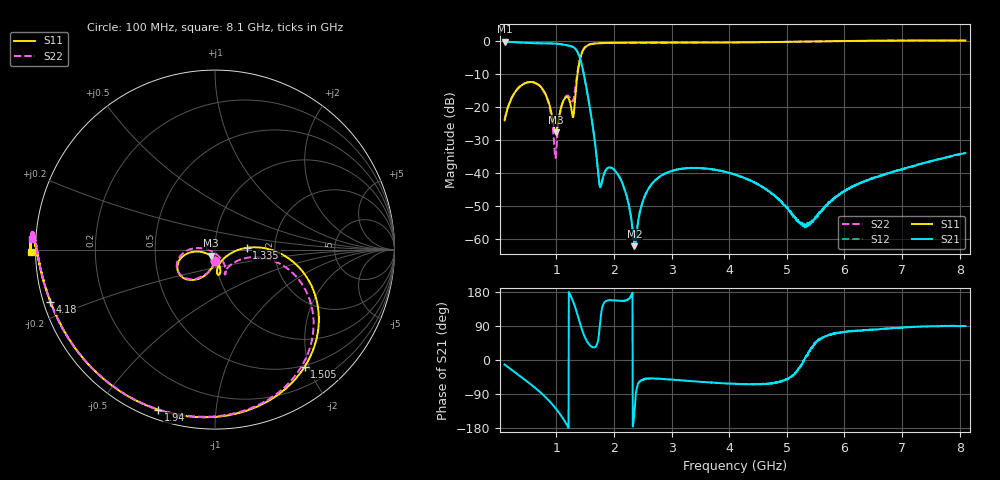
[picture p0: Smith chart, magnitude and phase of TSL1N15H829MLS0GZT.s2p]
! TSL1N15H829MLS0GZT  S-PARAMETER MODEL  ( General Type )
! Model Generated by TAIYO YUDEN Corporation (https://www.yuden.co.jp/en/)
! Version 1.0
! TAIYO YUDEN Control No. 210618
! Copyright(c) 2021 TAIYO YUDEN CO.,LTD. All Rights Reserved.
! Products Name : Multilayer Ceramic Devices
! Characteristics :
!  Passband freq : 617-960MHz ( At Passband , Insertion Loss : 0.95dB , VSWR 2.0 ),
!  Attenuation : 13dB min at 1554-1610MHz , 30dB min at 1710-2700MHz , Impedance : 50 Ohm ,
!  Case Size : 1.0 x 0.5 / 0.039 x 0.02 [mm/inch] , Thickness : 0.4 / 0.016 [mm/inch]
!  (Conditions: Temperature = 25 degC , DC Bias Current/Voltage = 0A / 0V)
! External Node Assignments :
!  1  o---|-------|---o  2
!  |  LPF  |
! GND o---|-------|---o GND
! Frequency Range : 100MHz  -  8.1GHz  [ 1601 STEP ]
# MHZ S RI R 50
! Freq[MHz].  S11 Real  S11 Imag  S21 Real  S21 Imag  S12 Real  S12 Imag  S22 Real  S22 Imag
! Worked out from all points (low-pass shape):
!   1601 points, 100 MHz to 8.1 GHz, reference 50 ohm
!   highest |S21| = -0.11 dB at 100 MHz (marker M1); lowest = -62.3 dB at 2.355 GHz (marker M2)
!   |S21| within 3 dB of the highest: start of sweep to 1.362 GHz
!   lowest |S11| = -27.7 dB at 985 MHz (marker M3), VSWR 1.09, Z = 47.7 - j3.29 ohm
!   |S11| at or under -10 dB: start of sweep to 1.366 GHz
!   |S22| runs from -35.5 to 0.2 dB; largest |S21 - S12| = 0.0013
!   S11 on the Smith chart (normalised r, x): 100 MHz: 0.99, -0.13; 1.335 GHz: 1.43, +0.03; 1.505 GHz: 0.48, -1.93; 1.94 GHz: 0.04, -0.71; 4.18 GHz: 0.02, -0.15; 8.1 GHz: -0.01, -0.01
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100  3.7e-05 -0.063  0.9663 -0.2038  0.9656 -0.2039  -0.00119 -0.064
325  -0.0949 -0.1636  0.762 -0.5889  0.762 -0.5887  -0.1 -0.161
645  -0.2094 -0.096  0.2353 -0.9018  0.236 -0.9018  -0.2129 -0.0822
845  -0.1325 -0.0145  -0.2142 -0.9051  -0.2141 -0.9054  -0.1279 0.00478
985  -0.0224 -0.0345  -0.5598 -0.7319  -0.5599 -0.732  -0.0061 -0.0155
1095  0.0288 -0.1051  -0.7785 -0.4489  -0.7786 -0.4485  0.0556 -0.0917
1200  0.0151 -0.1382  -0.8625 -0.0582  -0.8624 -0.058  0.0544 -0.1386
1280  0.0375 -0.0628  -0.7639 0.3097  -0.7638 0.3095  0.084 -0.0881
1335  0.1772 0.00997  -0.5324 0.5404  -0.5325 0.5405  0.2153 -0.0422
1435  0.5679 -0.2906  0.0483 0.4503  0.0479 0.4506  0.5459 -0.3583
1505  0.5002 -0.6516  0.1276 0.1926  0.1278 0.1926  0.4538 -0.6931
1750  -0.0811 -0.9339  0.000663 0.00639  0.000642 0.00639  -0.1196 -0.9293
1940  -0.3168 -0.8921  -0.0112 0.00451  -0.0111 0.00458  -0.3488 -0.8794
2185  -0.4921 -0.8122  -0.00508 0.00219  -0.00516 0.00215  -0.518 -0.7954
2355  -0.5726 -0.7589  -0.000511 -0.000575  -0.000629 -0.000537  -0.5952 -0.7405
2530  -0.6354 -0.7085  0.00274 -0.00328  0.00276 -0.00338  -0.6553 -0.6888
2770  -0.701 -0.6432  0.00548 -0.00645  0.00548 -0.00647  -0.7193 -0.6247
4100  -0.9081 -0.3101  0.00434 -0.00835  0.0043 -0.00833  -0.9138 -0.3009
4180  -0.9169 -0.2894  0.00401 -0.00793  0.00399 -0.00787  -0.9208 -0.2811
5435  -0.9914 -0.00907  0.00157 0.00106  0.00153 0.000963  -0.9921 -0.0028
6770  -1.02 0.0651  0.00122 0.00984  0.00107 0.0099  -1.017 0.099
8100  -1.025 -0.0131  0.000112 0.02  4.19e-05 0.02  -1.022 0.0605
